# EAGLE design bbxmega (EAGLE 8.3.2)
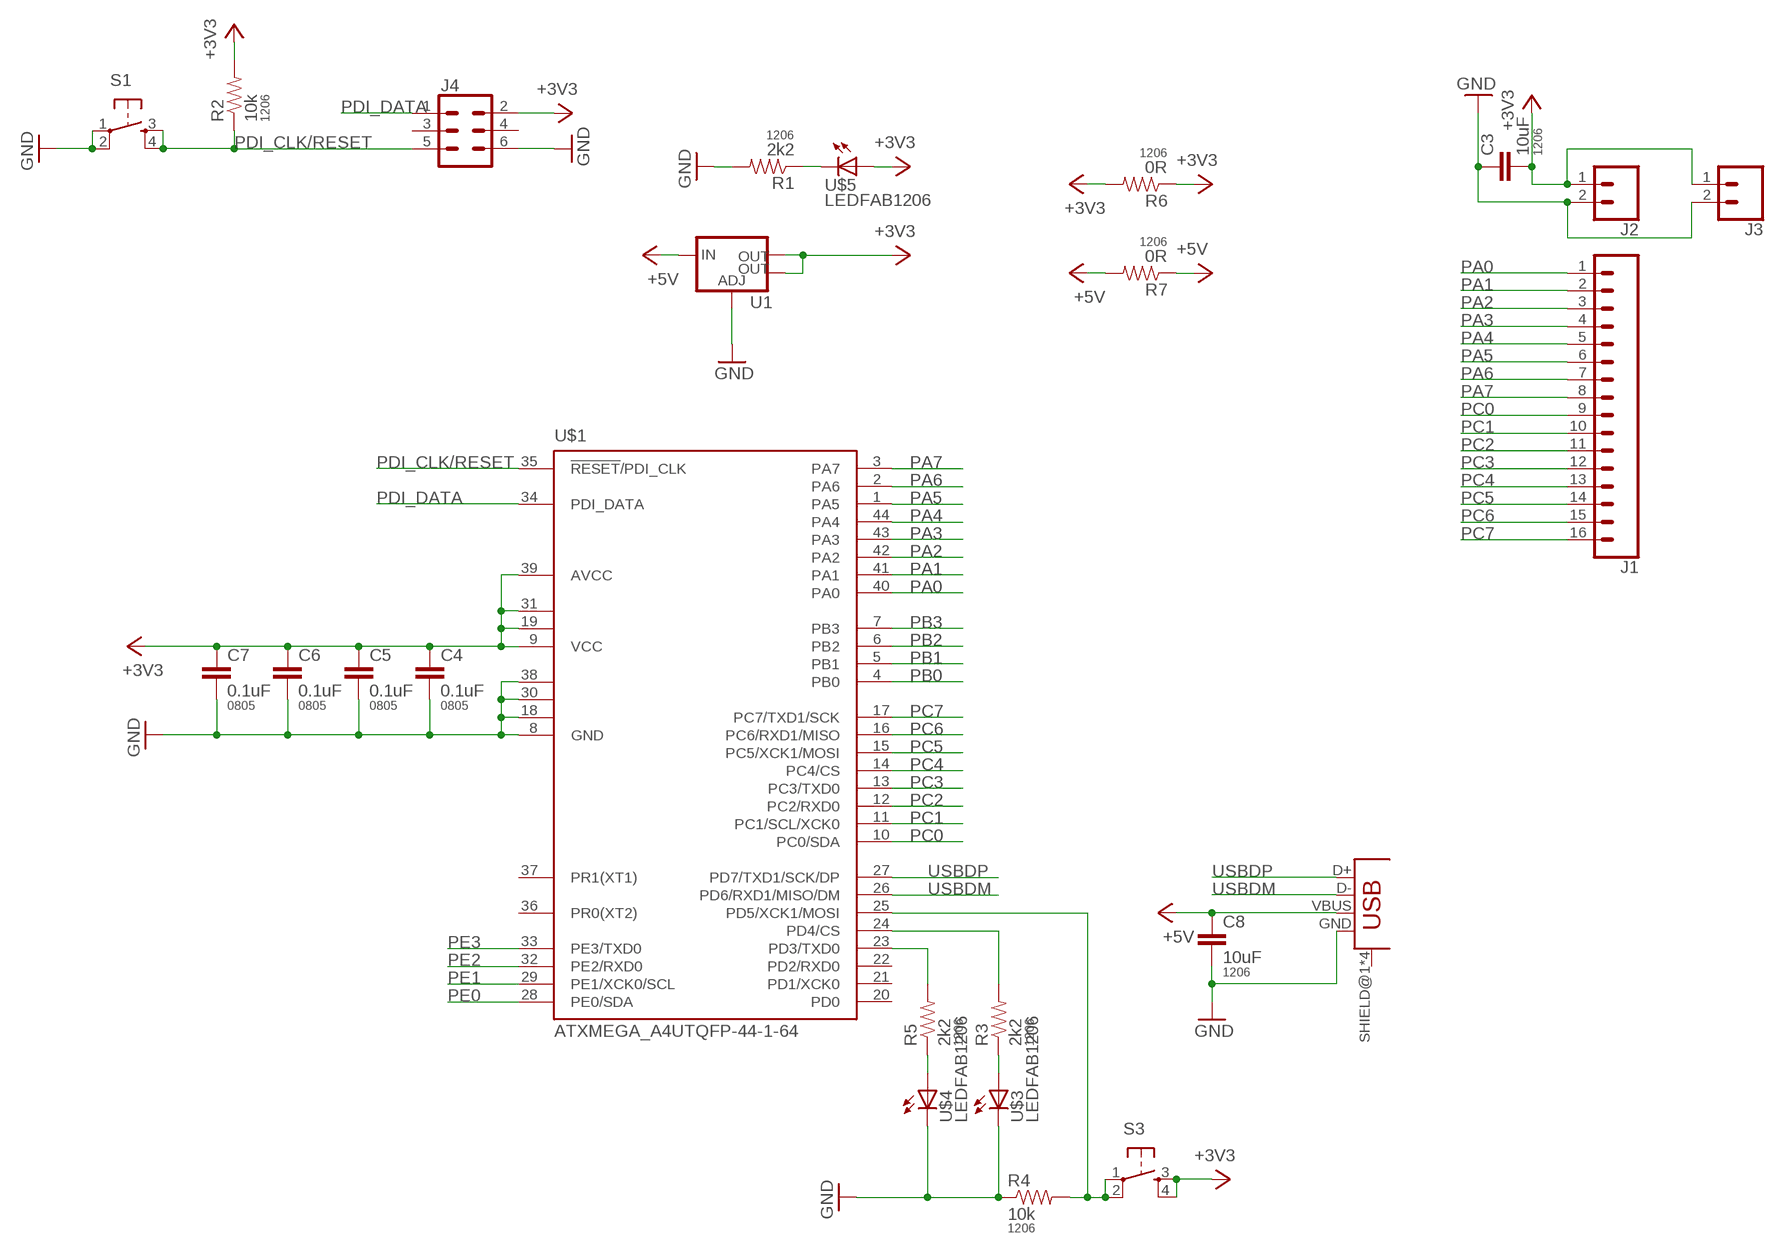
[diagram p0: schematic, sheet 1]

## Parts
C3  10uF  CAP1206  [1206]
C4  0.1uF  CAP0805  [0805]
C5  0.1uF  CAP0805  [0805]
C6  0.1uF  CAP0805  [0805]
C7  0.1uF  CAP0805  [0805]
C8  10uF  CAP1206  [1206]
J1  CONN_161X16_NO_SILK  [1X16_NO_SILK]
J2  CONN_02  [1X02]
J3  CONN_02  [1X02]
J4  CONN_03X2FEMALE_SMD  [2X3_SMD]
R1  2k2  RESISTOR1206  [1206]
R2  10k  RESISTOR1206  [1206]
R3  2k2  RESISTOR1206  [1206]
R4  10k  RESISTOR1206  [1206]
R5  2k2  RESISTOR1206  [1206]
R6  0R  RESISTOR1206  [1206]
R7  0R  RESISTOR1206  [1206]
S1  6MM_SWITCH6MM_SWITCH  [6MM_SWITCH]
S3  6MM_SWITCH6MM_SWITCH  [6MM_SWITCH]
U1  V_REG_LM1117SOT223  [SOT223]
U$1  ATXMEGA_A4UTQFP-44-1-64  [TQFP44-13THIN]
U$3  LEDFAB1206  [LED1206FAB]
U$4  LEDFAB1206  [LED1206FAB]
U$5  LEDFAB1206  [LED1206FAB]
X1  USB_MINIB  [USB_MINIB]

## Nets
+3V3: C3.2 C4.1 C5.1 C6.1 C7.1 J2.1 J3.1 J4.2 R2.2 R6.1 R6.2 S3.3(S) S3.4(S1) U1.2(OUT) U1.4(OUT) U$1.9(VCC) U$1.19(VCC1) U$1.31(VCC2) U$1.39(AVCC) U$5.1(A)
+5V: C8.1 R7.1 R7.2 U1.3(IN) X1.VBUS
GND: C3.1 C4.2 C5.2 C6.2 C7.2 C8.2 J2.2 J3.2 J4.6 R1.2 R4.1 S1.1(P) S1.2(P1) U1.1(ADJ) U$1.8(GND) U$1.18(GND1) U$1.30(GND2) U$1.38(GND3) U$3.2(C) U$4.2(C) X1.GND
N$1: R4.2 S3.1(P) S3.2(P1) U$1.25(PD5/XCK1/MOSI)
N$2: R3.2 U$1.24(PD4/CS)
N$3: R5.2 U$1.23(PD3/TXD0)
N$4: R5.1 U$4.1(A)
N$5: R3.1 U$3.1(A)
N$6: R1.1 U$5.2(C)
PA0: J1.1 U$1.40(PA0)
PA1: J1.2 U$1.41(PA1)
PA2: J1.3 U$1.42(PA2)
PA3: J1.4 U$1.43(PA3)
PA4: J1.5 U$1.44(PA4)
PA5: J1.6 U$1.1(PA5)
PA6: J1.7 U$1.2(PA6)
PA7: J1.8 U$1.3(PA7)
PB0: U$1.4(PB0)
PB1: U$1.5(PB1)
PB2: U$1.6(PB2)
PB3: U$1.7(PB3)
PC0: J1.9 U$1.10(PC0/SDA)
PC1: J1.10 U$1.11(PC1/SCL/XCK0)
PC2: J1.11 U$1.12(PC2/RXD0)
PC3: J1.12 U$1.13(PC3/TXD0)
PC4: J1.13 U$1.14(PC4/CS)
PC5: J1.14 U$1.15(PC5/XCK1/MOSI)
PC6: J1.15 U$1.16(PC6/RXD1/MISO)
PC7: J1.16 U$1.17(PC7/TXD1/SCK)
PDI_CLK/RESET: J4.5 R2.1 S1.3(S) S1.4(S1) U$1.35(!RESET!/PDI_CLK)
PDI_DATA: J4.1 U$1.34(PDI_DATA)
PE0: U$1.28(PE0/SDA)
PE1: U$1.29(PE1/XCK0/SCL)
PE2: U$1.32(PE2/RXD0)
PE3: U$1.33(PE3/TXD0)
USBDM: U$1.26(PD6/RXD1/MISO/DM) X1.D-
USBDP: U$1.27(PD7/TXD1/SCK/DP) X1.D+
Unconnected: J4.3 J4.4 U$1.20(PD0) U$1.21(PD1/XCK0) U$1.22(PD2/RXD0) U$1.36(PR0(XT2)) U$1.37(PR1(XT1)) X1.SHIELD@1(SHIELD) X1.SHIELD@2(SHIELD) X1.SHIELD@3(SHIELD) X1.SHIELD@4(SHIELD)

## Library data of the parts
C3 C8 = borkedlabs-passives:CAP: Capacitor; PACKAGE: 1206
C4-C7 = borkedlabs-passives:CAP: Capacitor; PACKAGE: 0805
J1 = SparkFun-Connectors:CONN_16: Multi connection point. Often used as Generic Header-pin footprint for 0.1 inch spaced/style header connections On any of the 0.1 inch spaced packages, you can populate with these: Break Away Headers - Straight (PRT-00116) Break Away Male Headers - Right Angle (PRT-00553) Female Headers (PRT-00115)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
J2 J3 = SparkFun-Connectors:CONN_02: Multi connection point. Often used as Generic Header-pin footprint for 0.1 inch spaced/style header connections
J4 = fab:CONN_03X2: Multi connection point. Often used as Generic Header-pin footprint for 0.1 inch spaced/style header connections You can populate with any combo of single row headers, but if you'd like an exact match, check these: Header - 2x3 (Male, 0.1") (PRT-12807) Header - 2x3 (Female, 0.1") (PRT-13010) 2x3 Pin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; PROD_ID: CONN-11290
R1-R7 = borkedlabs-passives:RESISTOR: Resistor; PACKAGE: 1206
S1 S3 = fab:6MM_SWITCH: OMRON SWITCH
U1 = fab:V_REG_LM1117: Voltage Regulator LM1117 Standard adjustable voltage regulator but in SMD form. Spark Fun Electronics SKU : COM-00595; PROD_ID: VREG-08170
U$1 = fab:ATXMEGA_A4U
U$3-U$5 = fab:LED: LED
X1 = fab:USB_MINIB

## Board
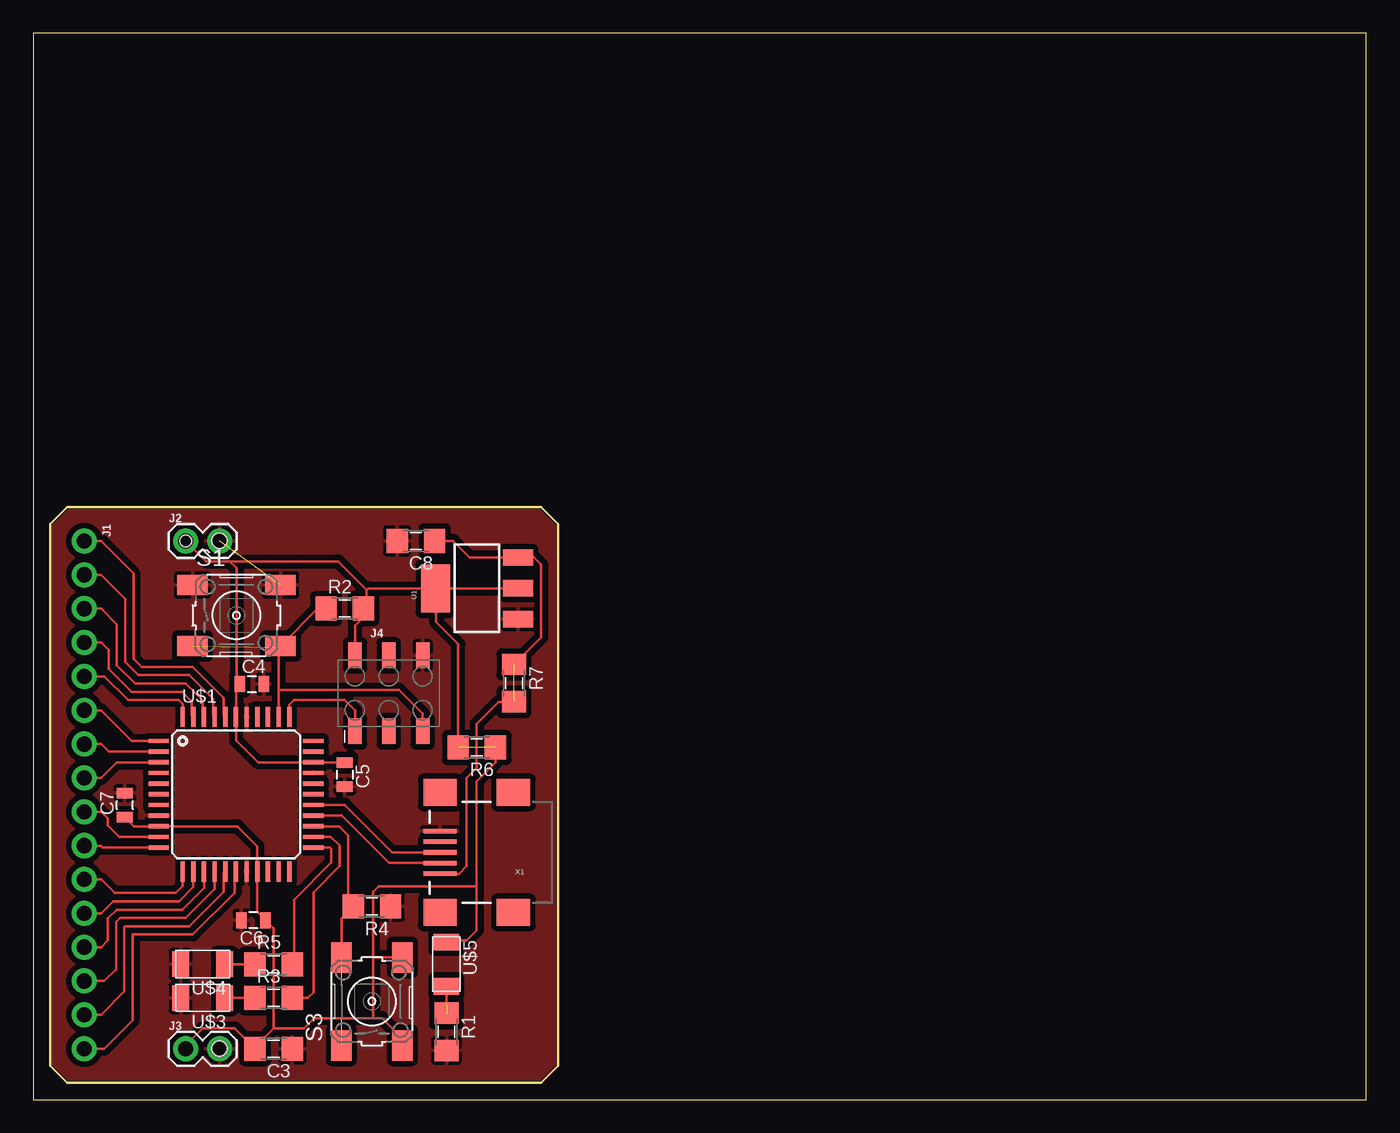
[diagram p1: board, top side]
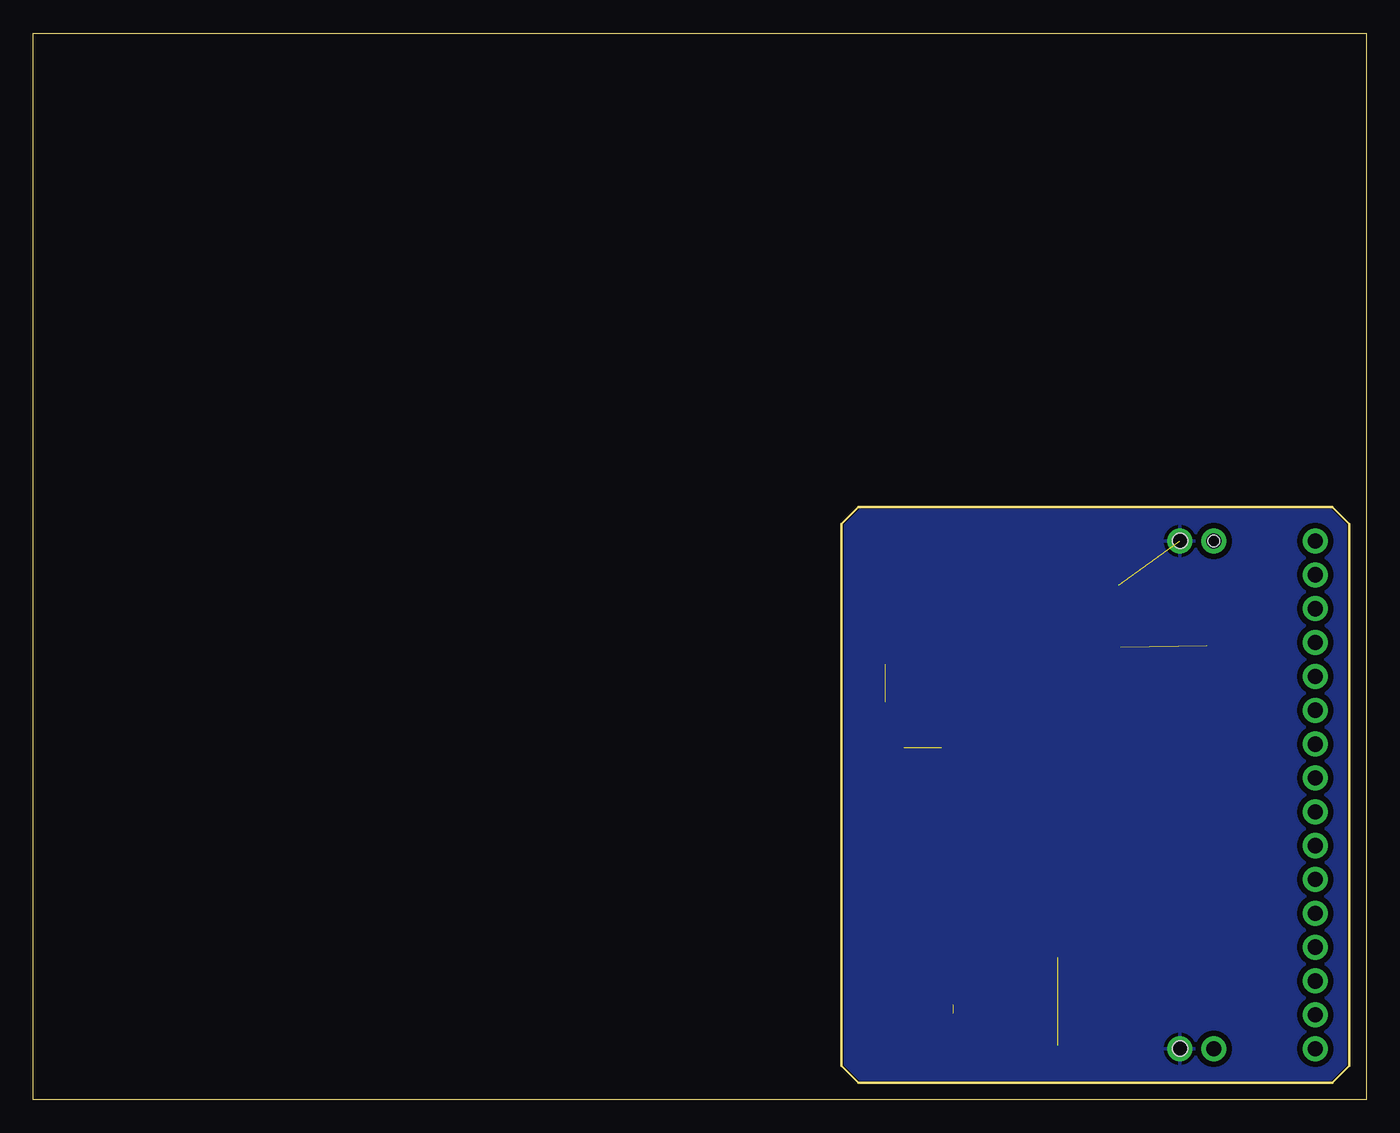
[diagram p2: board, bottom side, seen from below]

Size 100 x 80 mm. Coordinates in mm from the lower left corner, seen from the top.
Outline: 0,0 100,0 100,80 0,80 0,0
Outline: 1.27,43.18 2.54,44.45 38.1,44.45 39.37,43.18 39.37,2.54 38.1,1.27 2.54,1.27 1.27,2.54 1.27,43.18
Copper layers (1*16): Top 0.035mm / dielectric 1.5mm / Bottom 0.035mm
Design rules "default *": minimum track width 8mil, minimum drill 81mil, track to track 16.5mil, track to pad 16.5mil, pad to pad 16.5mil, via to via 16.5mil, smd to smd 6mil, copper to edge 2mil, drill to drill 6mil, minimum pad ring 10mil, minimum via ring 8mil, stop-mask expansion 4mil, vias tented up to drill 0mil, thermal gap 10mil
Holes 1.14 mm at 13.97,41.91 13.97,3.81
Holes 0.9 mm at 11.43,41.91

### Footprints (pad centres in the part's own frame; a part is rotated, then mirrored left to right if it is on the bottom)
1206 = smd 1.6 x 1.8: 1 -1.4,0; 2 1.4,0
0805 = smd 0.8 x 1.2: 1 -0.9,0; 2 0.9,0
1X16_NO_SILK = drill 1.143 pad 1.88: 1 0,0; 2 2.54,0; 3 5.08,0; 4 7.62,0; 5 10.16,0; 6 12.7,0; 7 15.24,0; 8 17.78,0; 9 20.32,0; 10 22.86,0; 11 25.4,0; 12 27.94,0; 13 30.48,0; 14 33.02,0; 15 35.56,0; 16 38.1,0
1X02 = drill 1.143 pad 1.88: 1 0,0; 2 2.54,0
2X3_SMD = smd 1.02 x 1.9: 1 -2.54,-2.85; 2 -2.54,2.85; 3 0,-2.85; 4 0,2.85; 5 2.54,-2.85; 6 2.54,2.85
6MM_SWITCH = smd 2.286 x 1.524: 1 -3.302,2.286; 2 3.302,2.286; 3 -3.302,-2.286; 4 3.302,-2.286
SOT223 = smd 1.219 x 2.235: 1 -2.311,-3.099; 2 0,-3.099; 3 2.311,-3.099 | smd 3.6 x 2.2: 4 0,3.099
TQFP44-13THIN = smd 1.524 x 0.33: 1 -5.8,4; 2 -5.8,3.2; 3 -5.8,2.4; 4 -5.8,1.6; 5 -5.8,0.8; 6 -5.8,0; 7 -5.8,-0.8; 8 -5.8,-1.6; 9 -5.8,-2.4; 10 -5.8,-3.2; 11 -5.8,-4; 23 5.8,-4; 24 5.8,-3.2; 25 5.8,-2.4; 26 5.8,-1.6; 27 5.8,-0.8; 28 5.8,0; 29 5.8,0.8; 30 5.8,1.6; 31 5.8,2.4; 32 5.8,3.2; 33 5.8,4 | smd 0.33 x 1.524: 12 -4,-5.8; 13 -3.2,-5.8; 14 -2.4,-5.8; 15 -1.6,-5.8; 16 -0.8,-5.8; 17 0,-5.8; 18 0.8,-5.8; 19 1.6,-5.8; 20 2.4,-5.8; 21 3.2,-5.8; 22 4,-5.8; 34 4,5.8; 35 3.2,5.8; 36 2.4,5.8; 37 1.6,5.8; 38 0.8,5.8; 39 0,5.8; 40 -0.8,5.8; 41 -1.6,5.8; 42 -2.4,5.8; 43 -3.2,5.8; 44 -4,5.8
LED1206FAB = smd 1.27 x 1.905: 1 -1.651,0; 2 1.651,0
USB_MINIB = smd 2.5 x 0.35: D+ 3.77,0; D- 3.77,0.8; GND 3.77,-1.6; ID 3.77,-0.8; VBUS 3.77,1.6 | smd 2.5 x 2: SHIELD@1 -1.73,-4.5; SHIELD@2 -1.73,4.5; SHIELD@3 3.77,4.5; SHIELD@4 3.77,-4.5

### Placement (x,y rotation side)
C3  18.03,3.81 180 top
C4  16.39,31.17 0 top
C5  23.37,24.38 270 top
C6  16.51,13.46 180 top
C7  6.86,22.1 90 top
C8  28.7,41.91 180 top
J1  3.81,41.91 270 top
J2  11.43,41.91 0 top
J3  11.43,3.81 0 top
J4  26.67,30.48 0 top
R1  30.99,5.08 270 top
R2  23.37,36.83 0 top
R3  18.03,7.62 0 top
R4  25.4,14.48 180 top
R5  18.03,10.16 0 top
R6  33.27,26.42 180 top
R7  36.07,31.24 270 top
S1  15.24,36.32 0 top
S3  25.4,7.37 90 top
U1  33.27,38.35 90 top
U$1  15.21,22.91 0 top
U$3  12.7,7.62 180 top
U$4  12.7,10.16 180 top
U$5  30.99,10.16 270 top
X1  34.29,18.54 180 top

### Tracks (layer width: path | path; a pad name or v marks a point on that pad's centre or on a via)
+3V3  (1 unrouted)
  Top 0.203: J3.1 11.43,4.06 12.7,5.33 15.11,5.33 16.57,3.87 | 16.57,3.87 C3.2 | S3.3 27.69,4.57 26.16,6.1 25.4,6.1 | 25.4,6.1 21.08,6.1 20.32,5.33 18.03,5.33 | 18.03,5.33 16.57,3.87 | S3.4 27.43,10.67 27.18,10.41 27.43,10.41 S3.4 | 24.87,36.78 25.21,36.64 | 24.87,36.78 R2.2 | 25.21,36.64 25.4,36.45 | 30.23,38.35 U1.2 | 30.23,38.35 U1.4 25.15,38.35 25.02,38.23 | J4.2 24.13,35.56 25.21,36.64 | J2.1 12.95,40.39 14.73,40.39 | 14.73,40.39 15.24,39.88 15.24,31.17 C4.1 15.21,30.89 U$1.39 15.21,26.96 16.86,25.31 U$1.31 23.34,25.31 C5.1 | C7.1 7.55,20.51 U$1.9 15.31,20.51 16.81,19.01 U$1.19 16.81,14.06 C6.1 18.03,12.84 18.03,5.33 | 14.73,40.39 22.87,40.39 25.02,38.23 | 25.02,38.23 25.02,36.93 24.87,36.78 | R6.2 31.87,34.17 30.23,35.81 30.23,38.35 | R6.1 34.67,25.28 33.27,23.88 33.27,16 | 33.27,16 33.27,12.7 32.51,11.94 31.11,11.94 U$5.1 | 33.27,16 25.89,16 25.48,15.59 25.48,10.67 | 25.4,6.1 25.48,6.17 25.48,10.67 | S3.4 25.48,10.67
+5V  (1 unrouted)
  Top 0.203: C8.1 31.5,41.91 32.74,40.66 U1.3 37.57,40.66 38.1,40.13 38.1,34.67 R7.1 | X1.VBUS 31.93,16.94 32.51,17.53 32.51,24.13 33.27,24.89 33.27,28.19 34.92,29.84 R7.2
GND  (1 unrouted)
  pour Top: 1.27,43.18 2.54,44.45 38.1,44.45 39.37,43.18 39.37,2.54 38.1,1.27 2.54,1.27 1.27,2.54
  pour Bottom: 1.27,43.18 2.54,44.45 38.1,44.45 39.37,43.18 39.37,2.54 38.1,1.27 2.54,1.27 1.27,2.54
N$1  (1 unrouted)
  Top 0.203: U$1.25 22.93,20.51 23.62,19.81 23.62,14.86 R4.2 23.11,13.59 S3.2
N$2
  Top 0.203: U$1.24 22.32,19.71 22.97,19.05 22.97,17.52 21.01,15.56 21.01,8.06 20.57,7.62 R3.2
N$3
  Top 0.203: 19.5,10.22 19.99,10.72 | 19.5,10.22 R5.2 | U$1.23 22.24,18.91 22.35,18.8 22.35,17.78 19.56,14.99 19.56,10.28 19.5,10.22
N$4
  Top 0.203: R5.1 U$4.1
N$5
  Top 0.203: R3.1 U$3.1
N$6  (1 unrouted)
  Top 0.203: U$5.2 30.99,7.11
PA0
  Top 0.203: U$1.40 14.29,28.82 14.29,30.12 11.95,32.46 8.14,32.46 7.53,33.07 7.53,39.46 5.08,41.91 J1.1
PA1
  Top 0.203: U$1.41 13.49,28.82 13.49,30.04 11.7,31.84 7.88,31.84 6.91,32.82 6.91,37.54 5.08,39.37 J1.2
PA2
  Top 0.203: U$1.42 12.69,28.82 12.69,29.96 11.44,31.22 7.63,31.22 6.27,32.58 6.27,35.64 5.08,36.83 J1.3
PA3
  Top 0.203: U$1.43 11.89,28.82 11.89,29.88 11.18,30.59 7.37,30.59 5.65,32.32 5.65,33.72 5.08,34.29 J1.4
PA4
  Top 0.203: J1.5 5.33,31.75 7.11,29.97 10.92,29.97 11.21,29.69 U$1.44
PA5
  Top 0.203: J1.6 5.08,29.21 7.38,26.91 U$1.1
PA6
  Top 0.203: J1.7 5.08,26.67 5.64,26.11 U$1.2
PA7
  Top 0.203: J1.8 5.08,24.13 6.26,25.31 U$1.3
PC0
  Top 0.203: J1.9 5.08,21.59 5.59,21.08 5.59,20.57 6.46,19.71 U$1.10
PC1
  Top 0.203: J1.10 5.08,19.05 5.22,18.91 U$1.11
PC2
  Top 0.203: U$1.12 11.21,16.03 10.67,15.49 6.1,15.49 5.08,16.51 J1.11
PC3
  Top 0.203: J1.12 5.08,13.97 5.98,14.87 10.93,14.87 12.01,15.95 U$1.13
PC4
  Top 0.203: J1.13 5.08,11.43 5.59,11.94 5.59,13.6 6.24,14.25 11.18,14.25 12.81,15.87 U$1.14
PC5
  Top 0.203: J1.14 5.33,8.89 6.21,9.77 6.21,13.32 6.51,13.63 11.44,13.63 13.61,15.79 U$1.15
PC6
  Top 0.203: J1.15 5.08,6.35 6.83,8.1 6.83,12.95 6.88,13.01 11.7,13.01 14.29,15.6 14.29,16.99 U$1.16
PC7
  Top 0.203: J1.16 5.33,3.81 7.46,5.93 7.46,12.38 11.96,12.38 15.09,15.52 15.09,16.99 U$1.17
PDI_CLK/RESET  (1 unrouted)
  Top 0.203: R2.1 21.34,36.83 S1.4 18.41,33.9 18.41,30.73 | 18.41,30.73 U$1.35 | J4.5 29.21,28.96 27.43,30.73 18.41,30.73
PDI_DATA
  Top 0.203: U$1.34 19.21,29.62 19.56,29.97 23.37,29.97 24.13,29.21 J4.1
USBDM
  Top 0.203: U$1.26 23.14,21.31 26.71,17.74 X1.D-
USBDP
  Top 0.203: U$1.27 23.36,22.11 26.92,18.54 X1.D+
